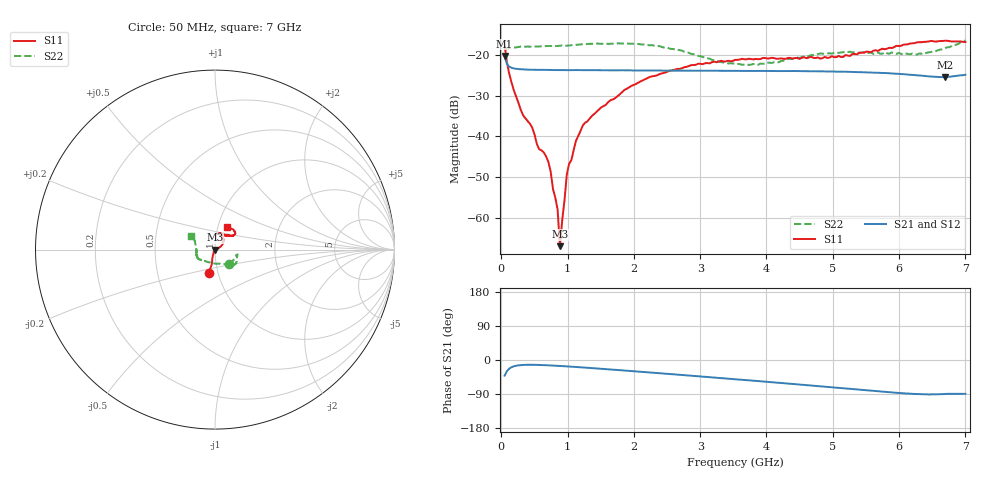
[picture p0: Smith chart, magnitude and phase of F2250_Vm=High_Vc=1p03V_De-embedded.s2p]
! Integrated Device Technology
! Corporate Headquarters
! 6024 Silver Creek Valley Road
! San Jose, CA 95138  USA
! Phone:  1-408-284-8200
! Toll Free:  1-800-223-1366
! Webpage:  http://www.idt.com/
! Timing and RF Division
! 515 Groton Road, Suite 102
! Westford, MA 01886-6024
! Device:  F2250
! Description: Voltage Variable RF Attenuator
! Frequency:  50.0 -  6000.00 MHz
! Package:  3x3 mm Thin QFN Plastic Package: 16 pin
! Ports:  2 RF, 3 DC
!  Pin  1  = GND
!  Pin  2  = NC
!  Pin  3  = RF1  = Port 1
!  Pin  4  = NC
!  Pin  5  = GND
!  Pin  6  = GND
!  Pin  7  = GND
!  Pin  8  = GND
!  Pin  9  = NC
!  Pin 10  = RF2  = Port 2
!  Pin 11  = NC
!  Pin 12  = GND
!  Pin 13  = GND
!  Pin 14  = VCNTRL
!  Pin 15  = VDD
!  Pin 16  = VMODE
! Vcntrl:  1.030 Volts
! Vmode:  +3.300 Volts
! Vdd:  +3.30  Volts
! Current:  1.328 mA
! Data:  The device was measured on a the F2250 evaluation board which has
!  individual transmission lines to the RF pins.  Data was collected
!  using a calibrated network analyzer.  The evaluation board was
!  de-embedded using a TRL calibration technique.
!  The reference plane is the edge of the package pin.
! Misc:  SN 10
!  Action Tracker AT0258
! Date Measured:  2014-11-26
! Date:  2015-10-15  MJV
! Note:
!  Integrated Device Technology supplies this data as a sample of measured
!  data at the package pin for this product.  Your particular data for this
!  product may vary.
!  Data was taken at 25 degrees C.
!  Integrated Device Technology reserves the right to change this data at anytime.
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# GHz S dB R 50
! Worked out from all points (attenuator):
!   201 points, 50 MHz to 7 GHz, reference 50 ohm
!   highest |S21| = -20.19 dB at 50 MHz (marker M1); lowest = -25.4 dB at 6.687 GHz (marker M2)
!   lowest |S11| = -67.1 dB at 884 MHz (marker M3), VSWR 1.00, Z = 50 - j0.0403 ohm
!   |S11| at or under -10 dB: start of sweep to end of sweep
!   |S22| runs from -22.4 to -16.3 dB; largest |S21 - S12| = 0.00022
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0.05  -17.31 -105.0  -20.19 -41.4  -20.20 -41.4  -18.83 -46.2
0.1195  -24.53 -105.1  -22.79 -22.9  -22.79 -22.9  -18.27 -17.4
0.29325  -33.41 -110.4  -23.44 -13.4  -23.43 -13.4  -17.85 -12.9
0.467  -37.82 -123.1  -23.56 -12.6  -23.55 -12.6  -17.90 -13.4
0.57125  -43.16 -129.1  -23.58 -13.0  -23.57 -13.0  -17.83 -15.6
0.71025  -46.30 -125.1  -23.60 -14.1  -23.59 -14.1  -17.70 -18.1
0.745  -48.70 -128.0  -23.63 -14.4  -23.63 -14.4  -17.70 -18.7
0.77975  -52.96 -143.0  -23.64 -14.7  -23.62 -14.7  -17.73 -19.3
0.84925  -58.02 -147.5  -23.63 -15.4  -23.63 -15.4  -17.69 -21.3
0.884  -67.07 -65.3  -23.64 -15.7  -23.65 -15.7  -17.64 -22.2
0.98825  -49.36 -25.1  -23.65 -16.8  -23.65 -16.8  -17.62 -23.8
1.12725  -41.04 7.4  -23.65 -18.3  -23.64 -18.4  -17.40 -25.9
1.2315  -37.22 12.5  -23.66 -19.6  -23.65 -19.6  -17.23 -27.9
1.857  -28.54 28.8  -23.71 -27.8  -23.72 -27.8  -17.07 -35.3
2.37825  -24.70 39.7  -23.75 -34.8  -23.76 -34.8  -17.72 -41.3
3.525  -21.13 68.5  -23.83 -50.7  -23.83 -50.8  -22.12 -86.9
3.8725  -20.95 74.8  -23.83 -55.6  -23.83 -55.6  -22.33 -110.9
4.7065  -20.64 70.3  -23.93 -68.0  -23.93 -68.0  -19.97 -145.5
5.85325  -18.14 38.9  -24.45 -85.1  -24.44 -85.2  -19.62 -166.7
6.3745  -16.69 39.7  -25.06 -90.7  -25.07 -90.8  -19.71 173.9
6.68725  -16.41 46.8  -25.40 -89.7  -25.40 -89.8  -18.29 157.0
7  -16.72 61.9  -24.80 -89.3  -24.81 -89.4  -16.34 150.2
